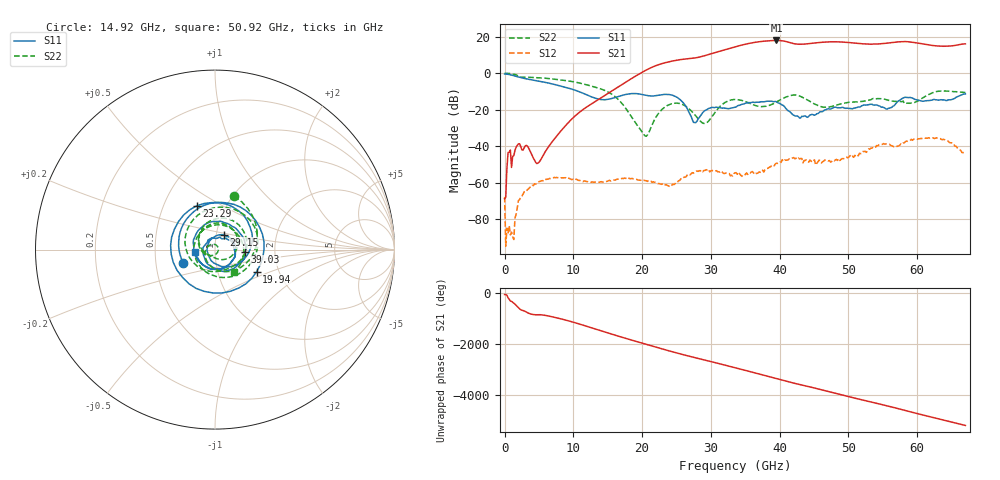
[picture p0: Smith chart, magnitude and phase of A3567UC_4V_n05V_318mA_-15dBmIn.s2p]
! MARKI MICROWAVE INC.
! Date:  4/20/2021
! Model Number:  A-3567UC
! Description:  2-port Small Signal S-parameter data for A-3567UC
! Frequency Range:  10 MHz to 67 GHz
! Port Configuration:  PORT 1: Input
!  PORT 2: Output
! Bias Condition: Vd = +4V, Vg = -0.5V, Id = 318mA
! A-3567UC s2p files are only valid for small signal conditions (below -10 dBm input power)
# Hz S  dB  R 50
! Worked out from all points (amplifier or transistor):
!   401 points, 10 MHz to 67 GHz, reference 50 ohm
!   highest |S21| = 18.0 dB at 39.53 GHz (marker M1)
!   |S21| within 3 dB of that: 34.01 GHz to 62.85 GHz (28.84 GHz wide, 59.5 % of centre)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
!   unconditionally stable (mu >= 1): 174.7 MHz to end of sweep
!   at 11.06 GHz: K = 3154.73, MAG = -19.0 dB, |S12| = -58.9 dB
!   at 33.51 GHz: K = 47.99, MAG = 14.7 dB, |S12| = -54.6 dB
!   at 67 GHz: K = 9.48, MAG = 16.8 dB, |S12| = -43.1 dB
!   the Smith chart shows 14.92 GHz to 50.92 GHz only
!   S11 on the Smith chart (normalised r, x): 14.92 GHz: 0.69, -0.10; 19.94 GHz: 1.54, -0.40; 23.29 GHz: 0.73, +0.38; 29.15 GHz: 1.09, +0.18; 39.03 GHz: 1.40, -0.04; 50.92 GHz: 0.80, -0.02
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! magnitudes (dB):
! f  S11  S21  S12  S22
! 10 MHz  -0.4  -68.7  -67.7  0.0
! 679.9 MHz  -0.7  -43.3  -83.5  -0.1
! 1.852 GHz  -1.9  -39.5  -73.7  -1.2
! 4.867 GHz  -4.2  -49.2  -59.7  -2.4
! 11.23 GHz  -10.7  -20.4  -59.0  -5.6
! 14.92 GHz  -14.3  -11.4  -59.2  -10.0
! 19.94 GHz  -11.6  0.4  -58.4  -31.9
! 20.78 GHz  -12.2  2.1  -59.3  -33.8
! 22.45 GHz  -12.0  4.8  -60.4  -21.7
! 23.29 GHz  -11.6  5.7  -61.3  -18.6
! 25.63 GHz  -14.8  7.5  -57.8  -16.8
! 27.64 GHz  -27.0  8.4  -54.0  -22.7
! 29.15 GHz  -20.4  9.7  -53.2  -27.4
! 33.51 GHz  -18.5  14.5  -54.6  -14.4
! 39.03 GHz  -15.5  17.9  -50.3  -16.8
! 39.53 GHz  -15.6  18.0  -49.3  -15.8
! 44.73 GHz  -22.5  16.5  -48.7  -16.1
! 50.92 GHz  -19.1  16.5  -45.0  -15.7
! 55.95 GHz  -19.1  16.7  -38.9  -15.0
! 58.29 GHz  -13.1  17.4  -37.5  -16.4
! 62.98 GHz  -14.7  15.0  -35.8  -9.9
! 67 GHz  -11.3  16.1  -43.1  -10.6
